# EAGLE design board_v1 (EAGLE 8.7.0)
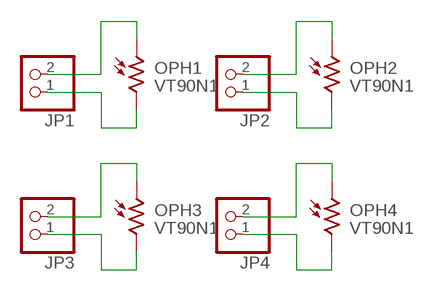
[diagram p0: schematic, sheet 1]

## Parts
JP1  PINHD-1X2  [1X02]
JP2  PINHD-1X2  [1X02]
JP3  PINHD-1X2  [1X02]
JP4  PINHD-1X2  [1X02]
OPH1  VT90N1  [VT900]
OPH2  VT90N1  [VT900]
OPH3  VT90N1  [VT900]
OPH4  VT90N1  [VT900]

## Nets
N$1: JP1.2 OPH1.1
N$2: JP1.1 OPH1.2
N$3: JP2.2 OPH2.1
N$4: JP2.1 OPH2.2
N$5: JP3.2 OPH3.1
N$6: JP3.1 OPH3.2
N$7: JP4.2 OPH4.1
N$8: JP4.1 OPH4.2

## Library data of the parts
JP1-JP4 = pinhead:PINHD-1X2: PIN HEADER
OPH1-OPH4 = photo-elements:VT9: Photoconductive Cell VT900 Series

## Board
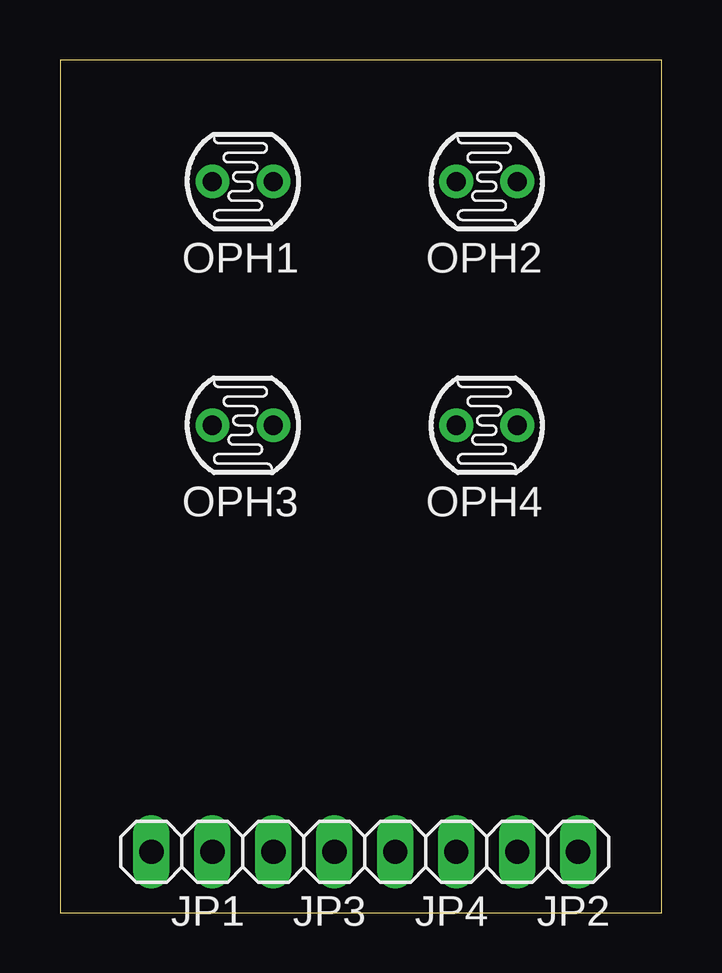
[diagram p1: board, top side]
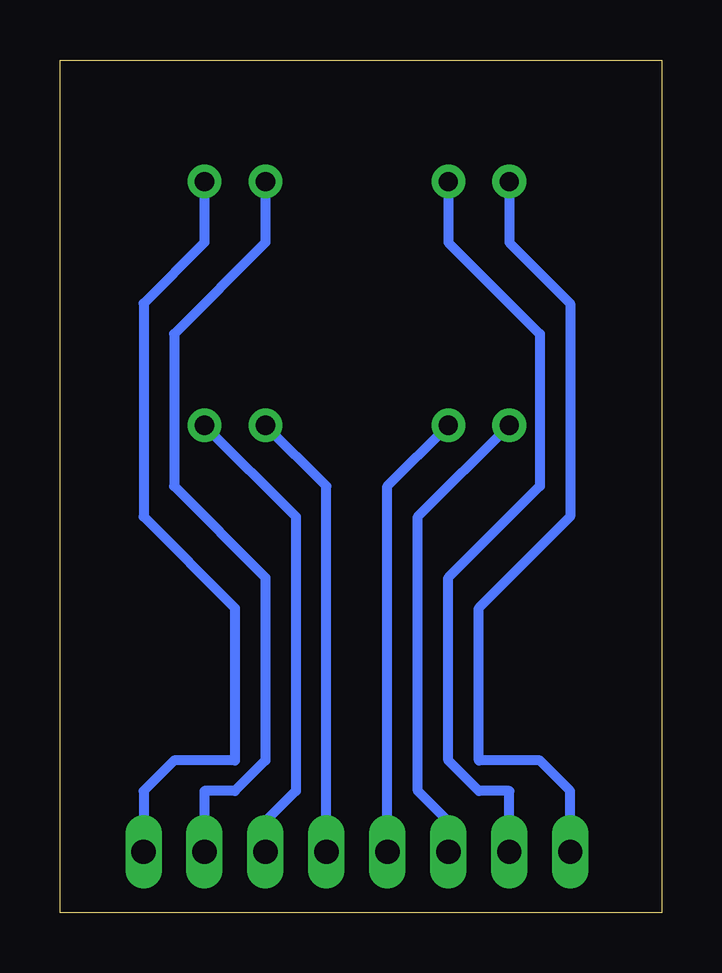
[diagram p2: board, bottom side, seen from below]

Size 25.07 x 35.55 mm. Coordinates in mm from the lower left corner, seen from the top.
Outline: 0,0 25.07,0 25.07,35.55 0,35.55 0,0
Copper layers (1*16): Top 0.035mm / dielectric 1.5mm / Bottom 0.035mm
Design rules "default": minimum track width 6mil, minimum drill 0.35mm, track to track 6mil, track to pad 6mil, pad to pad 6mil, via to via 6mil, smd to smd 6mil, copper to edge 40mil, drill to drill 6mil, minimum pad ring 10mil, minimum via ring 8mil, stop-mask expansion 4mil, vias tented up to drill 0mil, thermal gap 10mil

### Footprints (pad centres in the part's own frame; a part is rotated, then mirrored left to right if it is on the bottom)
1X02 = drill 1.016 long: 1 -1.27,0; 2 1.27,0
VT900 = drill 0.8 pad 1.4: 1 -1.27,0; 2 1.27,0

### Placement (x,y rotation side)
JP1  5.08,2.54 180 top
JP2  20.32,2.54 180 top
JP3  10.16,2.54 180 top
JP4  15.24,2.54 180 top
OPH1  7.62,30.48 0 top
OPH2  17.78,30.48 0 top
OPH3  7.62,20.32 0 top
OPH4  17.78,20.32 0 top

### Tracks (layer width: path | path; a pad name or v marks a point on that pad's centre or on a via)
N$1
  Bottom 0.406: OPH1.1 6.35,27.94 3.81,25.4 3.81,16.51 7.62,12.7 7.62,6.35 5.08,6.35 3.81,5.08 JP1.2
N$2
  Bottom 0.406: OPH1.2 8.89,27.94 5.08,24.13 5.08,17.78 8.89,13.97 8.89,6.35 7.62,5.08 6.35,5.08 JP1.1
N$3
  Bottom 0.406: OPH2.1 16.51,27.94 20.32,24.13 20.32,17.78 16.51,13.97 16.51,6.35 17.78,5.08 19.05,5.08 JP2.2
N$4
  Bottom 0.406: OPH2.2 19.05,27.94 21.59,25.4 21.59,16.51 17.78,12.7 17.78,6.35 20.32,6.35 21.59,5.08 JP2.1
N$5
  Bottom 0.406: OPH3.1 10.16,16.51 10.16,5.08 8.89,3.81 JP3.2
N$6
  Bottom 0.406: OPH3.2 11.43,17.78 JP3.1
N$7
  Bottom 0.406: OPH4.1 13.97,17.78 JP4.2
N$8
  Bottom 0.406: OPH4.2 15.24,16.51 15.24,5.08 16.51,3.81 JP4.1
